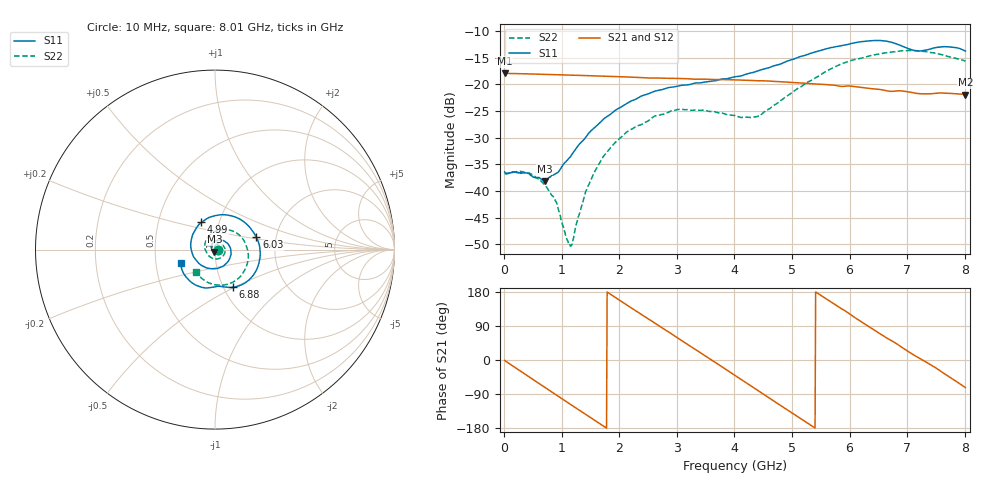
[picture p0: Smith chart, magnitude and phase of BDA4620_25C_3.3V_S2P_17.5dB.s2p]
!Agilent Technologies,E5071B,MY42404982,A.09.10
!Date: Wed May 06 08:52:24 2026
!Data & Calibration Information:
!Freq	S11:SOLT2(ON)	S21:SOLT2(ON)	S12:SOLT2(ON)	S22:SOLT2(ON)
# Hz S RI R 50
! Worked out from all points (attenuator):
!   801 points, 10 MHz to 8.01 GHz, reference 50 ohm
!   highest |S21| = -17.92 dB at 10 MHz (marker M1); lowest = -21.9 dB at 8.01 GHz (marker M2)
!   lowest |S11| = -38.1 dB at 710 MHz (marker M3), VSWR 1.03, Z = 49.7 - j1.2 ohm
!   |S11| at or under -10 dB: start of sweep to end of sweep
!   |S22| runs from -50.3 to -13.7 dB; largest |S21 - S12| = 0.00054
!   S11 on the Smith chart (normalised r, x): 10 MHz: 1.03, -0.00; 4.99 GHz: 0.82, +0.26; 6.03 GHz: 1.58, +0.23; 6.88 GHz: 1.10, -0.49; 8.01 GHz: 0.67, -0.11
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1e7  0.0151 -0.00104  0.127 -0.00273  0.1272 -0.00275  0.0145 -0.000515
4.4e8  0.00856 -0.0116  0.0883 -0.0886  0.0884 -0.0887  0.0136 -0.00569
7.1e8  -0.00324 -0.012  0.0375 -0.1182  0.0375 -0.1184  0.00825 -0.00788
8.9e8  -0.0118 -0.00837  -0.00112 -0.1232  -0.00132 -0.1234  0.00342 -0.0074
1.14e9  -0.0199 0.00524  -0.053 -0.11  -0.0531 -0.1101  -0.00254 -0.00193
1.19e9  -0.0206 0.00898  -0.0623 -0.1045  -0.0625 -0.1047  -0.00336 -0.000188
1.35e9  -0.0204 0.0207  -0.0883 -0.0828  -0.0884 -0.0829  -0.00508 0.00525
1.58e9  -0.0116 0.0378  -0.1125 -0.0414  -0.1126 -0.0415  -0.00416 0.0148
1.87e9  0.0126 0.0521  -0.1171 0.0179  -0.1173 0.018  0.00404 0.0259
2.68e9  0.0879 0.000921  -0.00247 0.1143  -0.00229 0.1144  0.0473 0.0193
3.41e9  0.0316 -0.0982  0.1056 0.0367  0.1057 0.0366  0.0446 -0.0358
4.01e9  -0.086 -0.0802  0.0834 -0.0717  0.0835 -0.0719  -0.0139 -0.049
4.42e9  -0.134 0.00815  0.0158 -0.1068  0.0157 -0.1069  -0.049 -0.0122
4.99e9  -0.0753 0.1519  -0.0784 -0.0688  -0.0785 -0.0689  -0.0345 0.0757
5.35e9  0.0332 0.1944  -0.1007 -0.00962  -0.1008 -0.00966  0.0242 0.1073
6.03e9  0.2309 0.0692  -0.0455 0.0845  -0.0456 0.0846  0.1572 0.0567
6.36e9  0.2473 -0.0657  0.00711 0.091  0.00713 0.0911  0.1845 -0.0167
6.68e9  0.1719 -0.1829  0.0496 0.0706  0.0497 0.0708  0.1737 -0.0972
6.88e9  0.0979 -0.2102  0.0699 0.0514  0.0701 0.0516  0.148 -0.1423
7.19e9  0.0192 -0.2038  0.0813 0.00932  0.0815 0.00935  0.0762 -0.1916
7.56e9  -0.0826 -0.2067  0.0737 -0.0379  0.0739 -0.038  -0.0203 -0.1905
8.01e9  -0.1907 -0.0749  0.0238 -0.0764  0.0239 -0.0765  -0.1086 -0.1241
